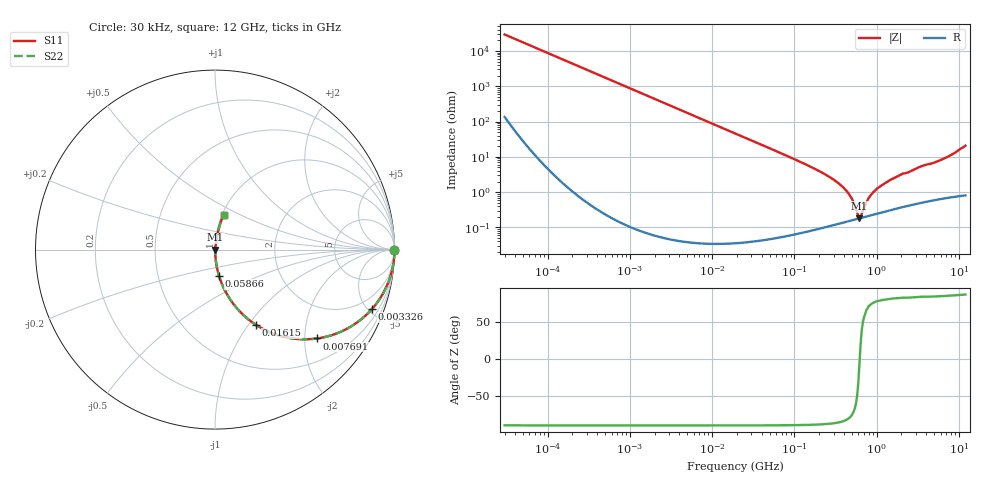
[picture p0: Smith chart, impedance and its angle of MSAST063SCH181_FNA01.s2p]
! MSAST063SCH181_FNA01  S-PARAMETER MODEL  ( Standard Model )
! Model Generated by TAIYO YUDEN Corporation (http://www.ty-top.com)
! Version 1.0
! TAIYO YUDEN Control No. 241122
! Copyright(c) 2024 TAIYO YUDEN CO.,LTD. All Rights Reserved.
! Product Description (link to TY-COMPAS)
! https://ds.yuden.co.jp/TYCOMPAS/or/detail?pn=MSAST063SCH181JFNA01&u=M
! Products Name : Multilayer Ceramic Capacitors
! Characteristics :
!  Capacitance : 180 [pF] , Rated Voltage : 25 [V] , TCC : CH / C0H
!  Case Size : 0.6 x 0.3 / 0.024 x 0.012 [mm/inch] , Thickness : 0.3 / 0.012 [mm/inch]
!  (Conditions: Temperature = 25 [degC] , DC Bias Voltage = 0 [V])
! External Node Assignments :
!  1  o---| |---o  2
! GND o---------o GND
! Frequency Range : 0.03MHz  -  12000MHz  [ 401 STEP ]
# MHZ S RI R 50
! Freq[MHz].  S11 Real  S11 Imag  S21 Real  S21 Imag  S12 Real  S12 Imag  S22 Real  S22 Imag
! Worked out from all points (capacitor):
!   401 points, 30 kHz to 12 GHz, reference 50 ohm
!   read as one part in series: C = 181 pF near 32 kHz
!   lowest |Z| = 182 mohm at 617.6 MHz (marker M1)
!   series resonance near 622 MHz, so ESL is about 360 pH
!   S11 on the Smith chart (normalised r, x): 30 kHz: open; 3.326 MHz: 1.00, -5.30; 7.691 MHz: 1.00, -2.29; 16.15 MHz: 1.00, -1.09; 58.66 MHz: 1.00, -0.30; 12 GHz: 1.02, +0.41
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0.03  1 -0.0034  2.72e-05 0.0034  2.72e-05 0.0034  1 -0.0034
0.260295  0.9991 -0.0295  0.000877 0.0295  0.000877 0.0295  0.9991 -0.0295
0.886466  0.99 -0.0995  0.01 0.0995  0.01 0.0995  0.99 -0.0995
2.258455  0.9384 -0.2404  0.0616 0.2404  0.0616 0.2404  0.9384 -0.2404
3.325624  0.8754 -0.3302  0.1246 0.3302  0.1246 0.3302  0.8754 -0.3302
7.691429  0.5677 -0.4952  0.4323 0.4952  0.4323 0.4952  0.5677 -0.4952
16.14825  0.2295 -0.4202  0.7705 0.4202  0.7705 0.4202  0.2295 -0.4202
18.97367  0.1775 -0.3817  0.8225 0.3817  0.8225 0.3817  0.1775 -0.3817
58.65857  0.0222 -0.1456  0.9778 0.1456  0.9778 0.1456  0.0222 -0.1456
164.6252  0.00329 -0.0496  0.9967 0.0496  0.9967 0.0496  0.00329 -0.0496
275.7901  0.00176 -0.0256  0.9982 0.0256  0.9982 0.0256  0.00176 -0.0256
393.2198  0.00155 -0.0134  0.9985 0.0134  0.9985 0.0134  0.00155 -0.0134
492.8008  0.00162 -0.00668  0.9984 0.00668  0.9984 0.00668  0.00162 -0.00668
579.0248  0.00174 -0.00207  0.9983 0.00207  0.9983 0.00207  0.00174 -0.00207
617.6002  0.00181 -0.000179  0.9982 0.000179  0.9982 0.000179  0.00181 -0.000179
658.7456  0.00189 0.00152  0.9981 -0.00152  0.9981 -0.00152  0.00189 0.00152
774.0045  0.00211 0.0054  0.9979 -0.0054  0.9979 -0.0054  0.00211 0.0054
880.5704  0.00233 0.00881  0.9977 -0.00881  0.9977 -0.00881  0.00233 0.00881
1428.372  0.00347 0.0212  0.9965 -0.0212  0.9965 -0.0212  0.00347 0.0212
3411.775  0.00761 0.052  0.9924 -0.052  0.9924 -0.052  0.00761 0.052
6715.658  0.0147 0.089  0.9853 -0.089  0.9853 -0.089  0.0147 0.089
12000  0.048 0.1951  0.952 -0.1951  0.952 -0.1951  0.048 0.1951
